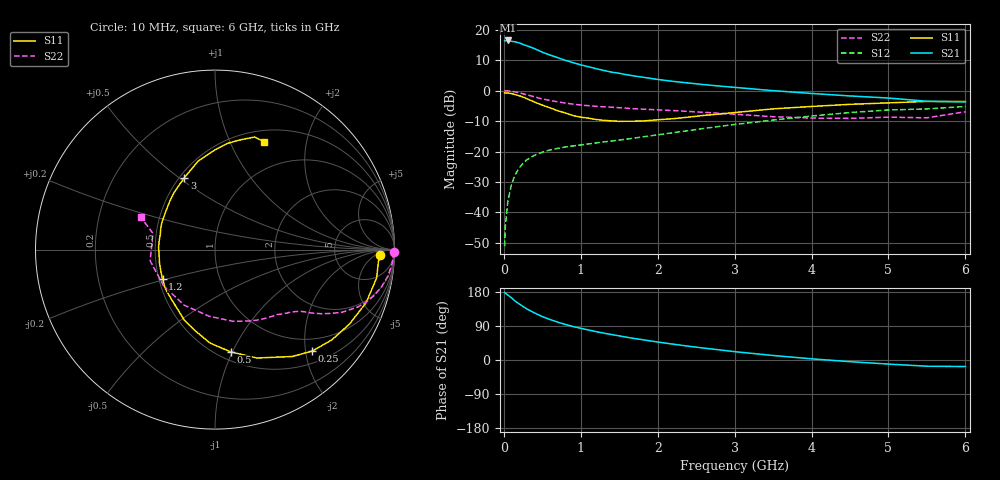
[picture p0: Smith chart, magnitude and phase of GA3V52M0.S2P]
! Infineon Technologies  Discrete & RF Semiconductors
! BF775
! Si NPN RF Bipolar Junction Transistor in SOT23
! VCE = 3.5 V  IC = 2 mA
! Common Emitter S-Parameters:  May  1996
# GHz  S  MA  R  50
!  f  S11  S21  S12  S22
! GHz  MAG  ANG  MAG  ANG  MAG  ANG  MAG  ANG
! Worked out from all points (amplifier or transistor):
!   36 points, 10 MHz to 6 GHz, reference 50 ohm
!   highest |S21| = 16.5 dB at 50 MHz (marker M1)
!   |S21| within 3 dB of that: start of sweep to 426.8 MHz
!   unconditionally stable (mu >= 1): 1.172 GHz to 3.719 GHz; 5.367 GHz to 5.816 GHz
!   at 250 MHz: K = 0.28, MSG = 19.5 dB, |S12| = -23.8 dB
!   at 1.4 GHz: K = 1.10, MAG = 9.4 dB, |S12| = -16.6 dB
!   at 6 GHz: K = 0.99, MSG = 0.7 dB, |S12| = -5.2 dB
!   S11 on the Smith chart (normalised r, x): 10 MHz: 21, -9; 250 MHz: 0.73, -2.14; 500 MHz: 0.58, -0.99; 1.2 GHz: 0.52, -0.20; 3 GHz: 0.53, +0.52; 6 GHz: 0.64, +1.36
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0.01  0.9218 -2.0  6.532 178.6  0.0028 90.0  0.9975 -0.8
0.02  0.9129 -4.1  6.569 176.5  0.0059 86.7  0.9921 -1.8
0.05  0.9143 -9.9  6.649 171.7  0.0147 82.7  0.9903 -4.5
0.1  0.8923 -19.4  6.444 163.9  0.0291 79.0  0.9742 -8.8
0.15  0.8566 -28.9  6.299 155.0  0.0421 73.1  0.9499 -12.8
0.2  0.8227 -37.7  6.065 148.0  0.0538 68.6  0.9195 -16.4
0.25  0.7832 -46.2  5.715 141.2  0.0642 64.0  0.887 -19.6
0.3  0.7352 -54.1  5.432 134.7  0.0734 60.7  0.8547 -22.1
0.4  0.6475 -68.9  4.877 124.2  0.0872 55.0  0.7885 -26.3
0.5  0.5768 -81.2  4.272 114.5  0.0975 50.8  0.73 -29.2
0.6  0.5221 -92.9  3.826 106.9  0.1061 47.9  0.6897 -31.2
0.8  0.4287 -113.5  3.142 93.8  0.1188 44.7  0.6245 -34.1
0.9  0.3894 -122.9  2.874 88.3  0.1237 44.6  0.5989 -35.2
1.1  0.3527 -141.5  2.463 79.2  0.1331 44.2  0.5649 -37.7
1.2  0.3358 -150.4  2.293 74.8  0.1385 44.1  0.5529 -39.0
1.6  0.3147 177.7  1.815 60.0  0.1601 45.5  0.5141 -44.4
2.2  0.3458 142.9  1.417 41.8  0.2036 47.3  0.4701 -55.2
3  0.4361 113.0  1.13 22.0  0.2777 44.6  0.4099 -76.5
3.5  0.5017 100.8  0.998 11.9  0.3288 40.3  0.3729 -95.0
4.5  0.5951 83.5  0.817 -4.4  0.4361 28.3  0.3503 -145.0
5.5  0.6647 70.6  0.669 -16.4  0.5 12.3  0.3576 165.3
6  0.6609 65.4  0.652 -17.2  0.5493 7.9  0.4497 156.5
